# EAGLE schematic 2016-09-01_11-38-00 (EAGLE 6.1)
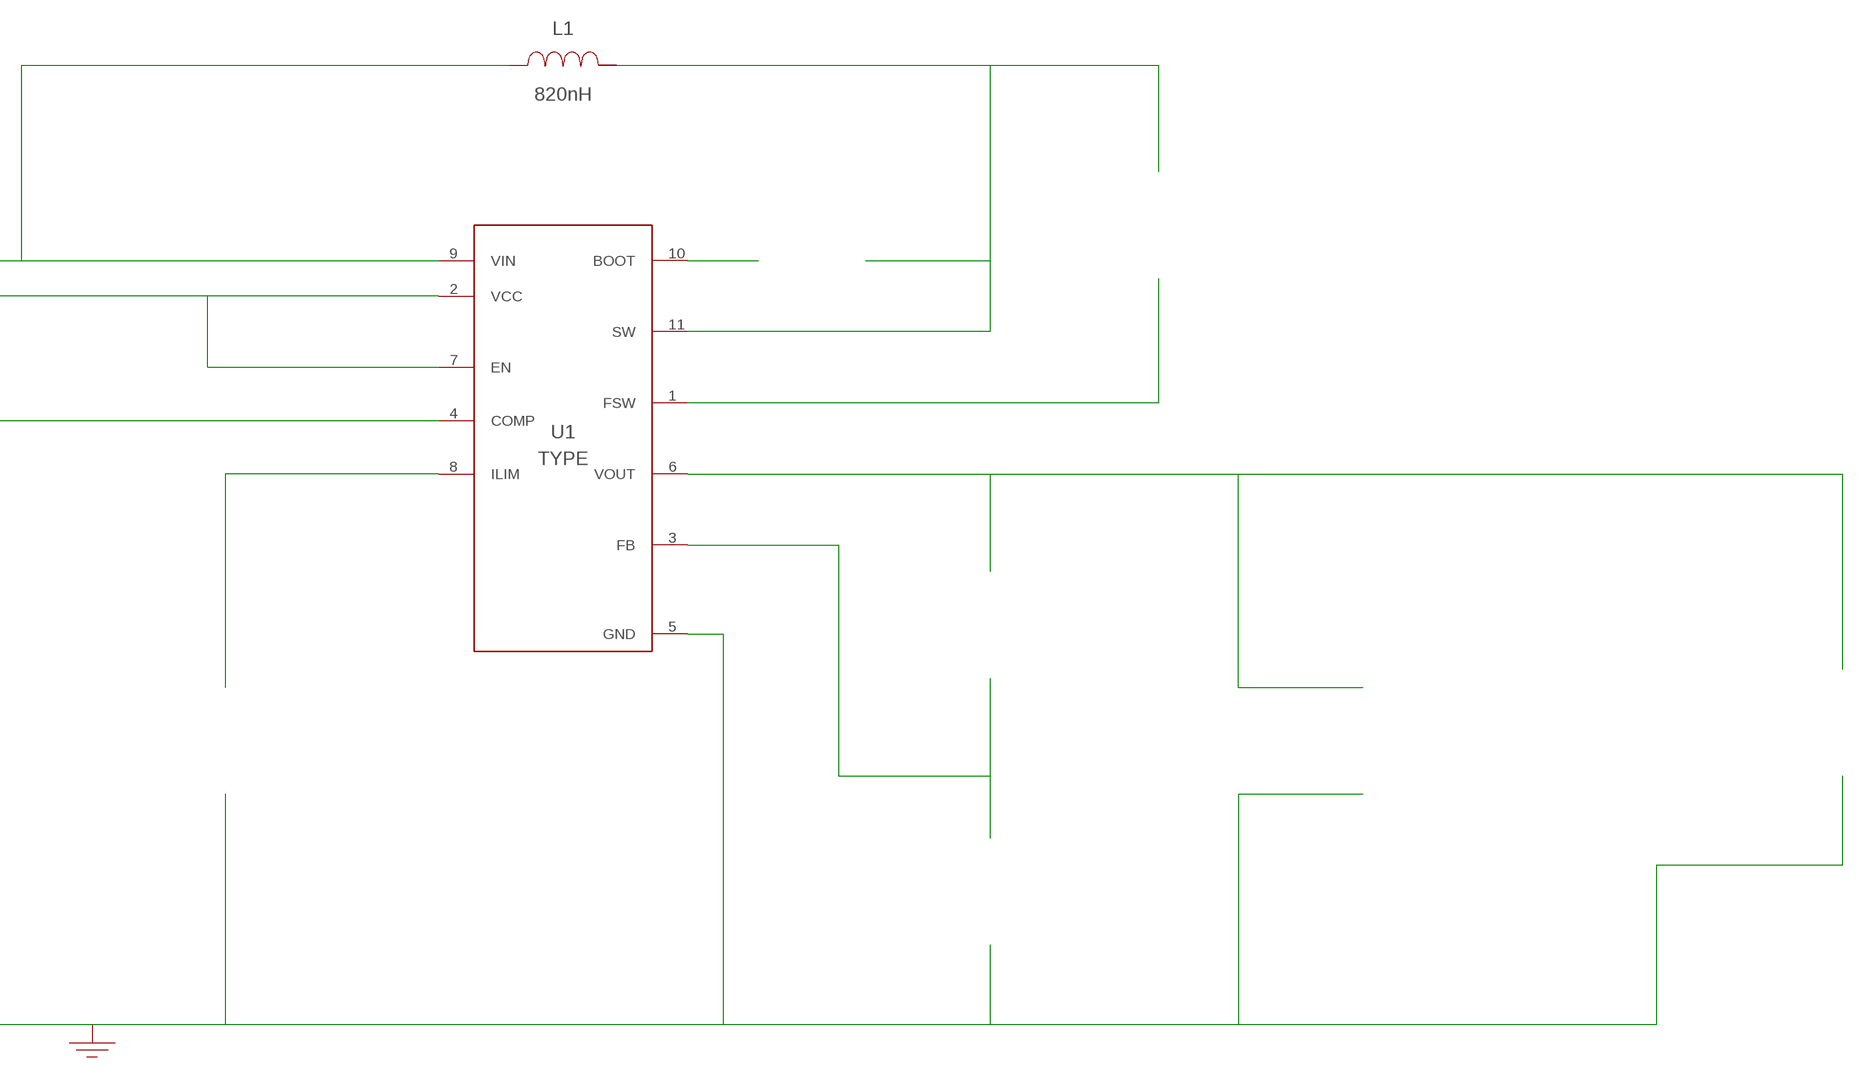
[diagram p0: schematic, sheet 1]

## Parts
CBST  100nF  GRM155R61A104KA01DGRM155R61A104KA01D  [0402]  (not placed on a sheet)
CCOMP  1.2nF  CL21C122JBFNNWECL21C122JBFNNWE  [0805]  (not placed on a sheet)
CCOMP2  62pF  CL21C620JBANNNCCL21C620JBANNNC  [0805]  (not placed on a sheet)
CIN  47uF  GRM31CR61A476KE15LGRM31CR61A476KE15L  [1206_190]  (not placed on a sheet)
CIN2  100nF  GRM155R60J104KA01DGRM155R60J104KA01D  [0402]  (not placed on a sheet)
CIN_2  47uF  GRM31CR61A476KE15LGRM31CR61A476KE15L  [1206_190]  (not placed on a sheet)
CIN_3  47uF  GRM31CR61A476KE15LGRM31CR61A476KE15L  [1206_190]  (not placed on a sheet)
COUT  47uF  GRM31CR61A476KE15LGRM31CR61A476KE15L  [1206_190]  (not placed on a sheet)
COUT_2  47uF  GRM31CR61A476KE15LGRM31CR61A476KE15L  [1206_190]  (not placed on a sheet)
CVCC  2.2uF  GRM188R61A225KE34DGRM188R61A225KE34D  [0603]  (not placed on a sheet)
GND1  WB_GND  WB_GNDWB_GND  [WB_GND]
IOUT  WB_CURRENT_LOAD  WB_CURRENT_LOADWB_CURRENT_LOAD  [WB_CURRENT_LOAD]  (not placed on a sheet)
L1  820nH  IHLP2020CZERR82M01IHLP2020CZERR82M01  [IHLP-2020CZ]
RCOMP  22.6k  CRCW040222K6FKEDCRCW040222K6FKED  [0402]  (not placed on a sheet)
RFBB  82k  RC0603FR-0782KLRC0603FR-0782KL  [0603]  (not placed on a sheet)
RFBT  243k  CRCW0402243KFKEDCRCW0402243KFKED  [0402]  (not placed on a sheet)
RLIM  143k  ERJ-8ENF1433VERJ-8ENF1433V  [1206]  (not placed on a sheet)
RT  523k  ERJ-8ENF5233VERJ-8ENF5233V  [1206]  (not placed on a sheet)
U1  TPS61089RNRR  TPS61089RNRRTPS61089RNRR  [RNR0011A]
VIN  WB_BATTERY  WB_BATTERYWB_BATTERY  [WB_BATTERY]  (not placed on a sheet)

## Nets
0: Ccomp2.2@2 Ccomp.2@2 Cin2.2@2 Cin.2@2 Cin_2.2@2 Cin_3.2@2 Cout.2@2 Cout_2.2@2 Cvcc.2@2 GND1.1 Iout.-@2 Rfbb.2@2 Rlim.2@2 U1.5(GND) Vin.-@2
1: Cin2.1@1 Cin.1@1 Cin_2.1@1 Cin_3.1@1 L1.1 U1.9(VIN) Vin.+@1
2: Cvcc.1@1 U1.2(VCC) U1.7(EN)
3: Ccomp2.1@1 Rcomp.1@1 U1.4(COMP)
4: Cout.1@1 Cout_2.1@1 Iout.+@1 Rfbt.1@1 U1.6(VOUT)
5: Ccomp.1@1 Rcomp.2@2
6: Rlim.1@1 U1.8(ILIM)
7: Rfbb.1@1 Rfbt.2@2 U1.3(FB)
8: Cbst.2@2 L1.2 Rt.1@1 U1.11(SW)
9: Rt.2@2 U1.1(FSW)
10: Cbst.1@1 U1.10(BOOT)
Unconnected: CBST.1 CBST.2 CCOMP2.1 CCOMP2.2 CCOMP.1 CCOMP.2 CIN2.1 CIN2.2 CIN.1 CIN.2 CIN_2.1 CIN_2.2 CIN_3.1 CIN_3.2 COUT.1 COUT.2 COUT_2.1 COUT_2.2 CVCC.1 CVCC.2 IOUT.1(+) IOUT.2(-) RCOMP.1 RCOMP.2 RFBB.1 RFBB.2 RFBT.1 RFBT.2 RLIM.1 RLIM.2 RT.1 RT.2 VIN.1(+) VIN.2(-)

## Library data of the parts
CBST = AcceleratedDesigns_Lib:GRM155R61A104KA01D; Cap: 1.0E-7; ESR: 0.0; IRMS: 0.0; Manufacturer_Name: MuRata; Manufacturer_Part_Number: GRM155R61A104KA01D; VDC: 10.0; Vendor: MuRata
CCOMP = AcceleratedDesigns_Lib:CL21C122JBFNNWE; Cap: 1.2E-9; Datasheet_URL: http://www.samsungsem.com/servlet/FileDownload?type%3Dspec%26file%3DCL21C122JBFNNWE.pdf; ESR: 0.0; IRMS: 0.0; Manufacturer_Name: Samsung Electro-Mechanics; Manufacturer_Part_Number: CL21C122JBFNNWE; VDC: 50.0; Vendor: Samsung Electro-Mechanics
CCOMP2 = AcceleratedDesigns_Lib:CL21C620JBANNNC; Cap: 6.2E-11; Datasheet_URL: http://www.samsungsem.com/servlet/FileDownload?type%3Dspec%26file%3DCL21C620JBANNNC.pdf; ESR: 0.0; IRMS: 0.0; Manufacturer_Name: Samsung Electro-Mechanics; Manufacturer_Part_Number: CL21C620JBANNNC; VDC: 50.0; Vendor: Samsung Electro-Mechanics
CIN CIN_2 CIN_3 COUT COUT_2 = AcceleratedDesigns_Lib:GRM31CR61A476KE15L; Cap: 4.7E-5; ESR: 0.0; IRMS: 0.0; Manufacturer_Name: MuRata; Manufacturer_Part_Number: GRM31CR61A476KE15L; VDC: 10.0; Vendor: MuRata
CIN2 = AcceleratedDesigns_Lib:GRM155R60J104KA01D; Cap: 1.0E-7; ESR: 0.0; IRMS: 0.0; Manufacturer_Name: MuRata; Manufacturer_Part_Number: GRM155R60J104KA01D; VDC: 6.3; Vendor: MuRata
CVCC = AcceleratedDesigns_Lib:GRM188R61A225KE34D; Cap: 2.2E-6; ESR: 0.0; IRMS: 0.0; Manufacturer_Name: MuRata; Manufacturer_Part_Number: GRM188R61A225KE34D; VDC: 10.0; Vendor: MuRata
GND1 = AcceleratedDesigns_Lib:WB_GND; Manufacturer_Name: WB_GND; Manufacturer_Part_Number: WB_GND; PowerPortType: POWER_GROUND; Value: Value
IOUT = AcceleratedDesigns_Lib:WB_CURRENT_LOAD; Manufacturer_Name: WB_CURRENT_LOAD; Manufacturer_Part_Number: WB_CURRENT_LOAD; PowerPortType: POWER_GROUND; Value: Value
L1 = AcceleratedDesigns_Lib:IHLP2020CZERR82M01; DCR: 11.9; Datasheet_URL: http://www.vishay.com/docs/34280/lp20cz01.pdf; Description: Unknown; IDC: 9.3; L: 8.2E-7; Manufacturer: Vishay; Manufacturer_Name: Vishay-Dale; Manufacturer_Part_Number: IHLP2020CZERR82M01; PACKAGE_DESIGNATOR: IHLP-2020CZ; Vendor: Vishay-Dale
RCOMP = AcceleratedDesigns_Lib:CRCW040222K6FKED; Manufacturer_Name: Vishay-Dale; Manufacturer_Part_Number: CRCW040222K6FKED; Power: 0.063; Resistance: 22600.0; Tolerance: 1.0; Vendor: Vishay-Dale
RFBB = AcceleratedDesigns_Lib:RC0603FR-0782KL; Manufacturer_Name: Yageo America; Manufacturer_Part_Number: RC0603FR-0782KL; Power: 0.1; Resistance: 82000.0; Tolerance: 1.0; Vendor: Yageo America
RFBT = AcceleratedDesigns_Lib:CRCW0402243KFKED; Manufacturer_Name: Vishay-Dale; Manufacturer_Part_Number: CRCW0402243KFKED; Power: 0.063; Resistance: 243000.0; Tolerance: 1.0; Vendor: Vishay-Dale
RLIM = AcceleratedDesigns_Lib:ERJ-8ENF1433V; Manufacturer_Name: Panasonic; Manufacturer_Part_Number: ERJ-8ENF1433V; Power: 0.25; Resistance: 143000.0; Tolerance: 1.0; Vendor: Panasonic
RT = AcceleratedDesigns_Lib:ERJ-8ENF5233V; Manufacturer_Name: Panasonic; Manufacturer_Part_Number: ERJ-8ENF5233V; Power: 0.25; Resistance: 523000.0; Tolerance: 1.0; Vendor: Panasonic
U1 = AcceleratedDesigns_Lib:TPS61089RNRR; Manufacturer: Texas Instruments; Manufacturer_Name: Texas Instruments; Manufacturer_Part_Number: TPS61089RNRR; PartNumber: TPS61089RNRR; RefDes: RefDes; TYPE: TYPE; Value: Value
VIN = AcceleratedDesigns_Lib:WB_BATTERY; Manufacturer_Name: WB_BATTERY; Manufacturer_Part_Number: WB_BATTERY; PowerPortType: POWER_GROUND; Value: Value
